|   stm32f427_437_429_439_wlcsp143 IBIS Model
[IBIS ver]   4.2
[File name]  stm32f427_437_429_439_wlcsp143.ibs
[File Rev]   1.3
[Date]   05-30-2014
[Source] Data Created at STMicroelectronics
[Notes]   File originated from ELDO simulations.
[Disclaimer]  This information is for modeling purpose only and is
   not guaranted. The information is subject to change without
   notice.
[Copyright] Copyright 2014 STMicroelectronics Inc.
[Component] stm32f427_437_429_439_wlcsp143
[Manufacturer] STMicroelectronics
[Package]
| variable   typ   min   max
R_pkg   0.0   NA   NA
L_pkg   0.0H   NA   NA
C_pkg   0.0F   NA   NA
[Pin]   signal_name   model_name  R_pin L_pin C_pin
A1   VDD  POWER
A10  PE1  io8p_arsudq_ft
A11  PDR_ON  io8p_arsudq_ft_v33
A2  PC10  io8p_arsudq_ft
A3  PD2  io8p_arsudq_ft
A4  PD5  io8p_arsudq_ft
A5  PD7  io8p_arsudq_ft
A6  PG12  io8p_arsudq_ft
A7  PG15  io8p_arsudq_ft
A8  PB6  io8p_arsudq_i2cin_ft
A9  PB8  io8p_arsudq_i2cin_ft
B1  PA14  io8p_arsudq_ft
B10  PE0  io8p_arsudq_ft
B11  PE4  io8p_arsudq_ft
B2  PC11  io8p_arsudq_ft
B3  PD0  io8p_arsudq_ft
B4  PD3  io8p_arsudq_ft
B5  PD4  io8p_arsudq_ft
B6  PG11  io8p_arsudq_ft
B7  PB3  io8p_arsudq_ft
B8  PB7  io8p_arsudq_i2cin_ft
B9  PB9  io8p_arsudq_i2cin_ft
C1  VDD  POWER
C10  PE3  io8p_arsudq_ft
C11  VBAT  POWER
C2  PA15  io8p_arsudq_ft
C3  PC12  io8p_arsudq_ft
C4  PD1  io8p_arsudq_ft
C5  VDD  POWER
C6  PG10  io8p_arsudq_ft
C7  PB4  io8p_arsudq_ft
C8  PB5  io8p_ar3wsudq_ft
C9  BOOT0  vpp_test_hv
D1   VCAP2  POWER
D10  PC13  io8p_arwsudq_ft_v33
D11  PC14  io8p_arwsudq_ft
D3  PA13  io8p_arsudq_ft
D4  PA11  io8usb_lsfs_otg_ft
D5  PA10  io8usb_id_otg_ft
D6  PG13  io8p_arsudq_ft
D7  VDD  POWER
D8  PE2  io8p_arsudq_ft
D9  PE5  io8p_arsudq_ft
E1  PA12  io8usb_lsfs_otg_ft
E10  VDD  POWER
E11  PC15  io8p_arsudq_ft
E2  PA9  io8usb_vbus_otg_ft
E3  PC9  io8p_arsudq_i2cin_ft
E4  PC8  io8p_arsudq_ft
E5  PG9  io8p_arsudq_ft
E6  VDD  POWER
E8  PE6  io8p_arsudq_ft
E9  PF1  io8p_arsudq_i2cin_ft
F1  PA8  io8p_arsudq_i2cin_ft
F10  PF2  io8p_arsudq_ft
F11  PF0  io8p_arsudq_i2cin_ft
F2  PC6  io8p_arsudq_ft
F3  PC7  io8p_arsudq_ft
F4  PD6  io8p_arsudq_ft
F6  PG14  io8p_arsudq_ft
F7  PF7  io8p_arwsudq_ft
F8  PF5  io8p_arwsudq_ft
F9  PF4  io8p_arwsudq_ft
G1  VDD  POWER
G10  PF6  io8p_arwsudq_ft
G11  PF3  io8p_arwsudq_ft
G2  PG8  io8p_arsudq_ft
G3  PG3  io8p_arsudq_ft
G4  PG6  io8p_arsudq_ft
G5  PG4  io8p_arsudq_ft
G6  PG5  io8p_arsudq_ft
G7  VDD  POWER
G8  PF9  io8p_arwsudq_ft
G9  PF10  io8p_arwsudq_ft
H1  PG7  io8p_arsudq_ft
H10  PH1  io8p_arsudq_ft
H11  PF8  io8p_arwsudq_ft
H4  PD10  io8p_arsudq_ft
H5  PD13  io8p_arsudq_ft
H6  PD12  io8p_arsudq_ft
H8  PC0  io8p_ar3wsudq_ft
H9  NRST  ioreset_ft_v33
J1  PG2  io8p_arsudq_ft
J10  PC2  io8p_ar3wsudq_ft
J11  PH0  io8p_arsudq_ft
J2  PD14  io8p_arsudq_ft
J3  PB15  io8usb_lsfs_otg_ft
J4  PE10  io8p_arsudq_ft
J5  VDD  POWER
J6  VDD  POWER
J7  VDD  POWER
J8  VDD  POWER
J9  PC3  io8p_ar3wsudq_ft_x2
K1   PD15  io8p_arsudq_ft
K10  VSSA  GND
| K11: io8p_combi = io8p_arsudq_ft_v33_c (PDR_ON) + io8p_ar3wsudq_ft_c (PC1)
K11  PC1   io8p_combi
K2  PD11  io8p_arsudq_ft
K3  PB14  io8usb_lsfs_otg_ft
K4  PE11  io8p_arsudq_ft
K5  PG1  io8p_arsudq_ft
K6  PF13  io8p_arsudq_ft
K7  PB1  io8p_ar3wsudq_ft
K8  PA1  io8p_ar3wsudq_ft
K9  PA0  io8p_ar3wsudq_ft_v33
L1   VDD  POWER
L10  VDDA  POWER
L11  VREF+  POWER
L2  PD8  io8p_arsudq_ft
L3  PE15  io8p_ar3wsudq_ft
L4  PE12  io8p_arsudq_ft
L5  PE7  io8p_arsudq_ft
L6  PF14  io8p_arsudq_ft
L7  PB2  io8p_ar3wsudq_ft
L8  PA7  io8p_ar3wsudq_ft
L9  PA2  io8p_ar3wsudq_ft
M1  PD9  io8p_arsudq_ft
M10  PA4  io8p_ar3wsudq_ft
M11  PA3  io8p_ar3wsudq_ft
M2  PB12  io8usb_id_otg_ft
M3  PB10  io8p_arsudq_i2cin_ft
M4  PE14  io8p_arsudq_ft
M5  PE8  io8p_arsudq_ft
M6  PF15  io8p_arsudq_ft
M7  PF11  io8p_arsudq_ft
M8  PC4  io8p_ar3wsudq_ft
M9  PA5  io8p_ar3wsudq_ft
N1  PB13  io8usb_vbus_otg_ft
N10  PA6  io8p_ar3wsudq_ft
N11  BYPASS_REG  io8p_arsudq_ft_v33
N2  VCAP1  POWER
N3  PB11  io8p_arsudq_i2cin_ft
N4  PE13  io8p_arsudq_ft
N5  PE9  io8p_arsudq_ft
N6  PG0  io8p_arsudq_ft
N7  PF12  io8p_arsudq_ft
N8  PB0  io8p_ar3wsudq_ft
N9  PC5  io8p_ar3wsudq_ft
[Diff Pin]   inv_pin   vdiff   tdelay_typ  tdelay_min  tdelay_max
D4   E1   200mV   NA   NA   NA
K1   J3   200mV   NA   NA   NA
[Model Selector] io8p_ar3wsudq_ft
io8p00_ar3wsudq_ft_pd_lv  "SPEED00 1P8V, PD=40kOhm"
io8p00_ar3wsudq_ft_pu_lv  "SPEED00 1P8V, PU=40kOhm"
io8p00_ar3wsudq_ft_lv  "SPEED00 1P8V"
io8p01_ar3wsudq_ft_pd_lv  "SPEED01 1P8V, PD=40kOhm"
io8p01_ar3wsudq_ft_pu_lv  "SPEED01 1P8V, PU=40kOhm"
io8p01_ar3wsudq_ft_lv  "SPEED01 1P8V"
io8p10_ar3wsudq_ft_pd_lv  "SPEED10 1P8V, PD=40kOhm"
io8p10_ar3wsudq_ft_pu_lv  "SPEED10 1P8V, PU=40kOhm"
io8p10_ar3wsudq_ft_lv  "SPEED10 1P8V"
io8p11_ar3wsudq_ft_pd_lv  "SPEED11 1P8V, PD=40kOhm"
io8p11_ar3wsudq_ft_pu_lv  "SPEED11 1P8V, PU=40kOhm"
io8p11_ar3wsudq_ft_lv  "SPEED11 1P8V"
io8p00_ar3wsudq_ft_pd  "SPEED00, PD=40kOhm"
io8p00_ar3wsudq_ft_pu  "SPEED00, PU=40kOhm"
io8p00_ar3wsudq_ft  "SPEED00"
io8p01_ar3wsudq_ft_pd  "SPEED01, PD=40kOhm"
io8p01_ar3wsudq_ft_pu  "SPEED01, PU=40kOhm"
io8p01_ar3wsudq_ft  "SPEED01"
io8p10_ar3wsudq_ft_pd  "SPEED10, PD=40kOhm"
io8p10_ar3wsudq_ft_pu  "SPEED10, PU=40kOhm"
io8p10_ar3wsudq_ft  "SPEED10"
io8p11_ar3wsudq_ft_pd  "SPEED11, PD=40kOhm"
io8p11_ar3wsudq_ft_pu  "SPEED11, PU=40kOhm"
io8p11_ar3wsudq_ft  "SPEED11"
[Model Selector] io8p_ar3wsudq_ft_v33
io8p00_ar3wsudq_ft_v33_pd_lv  "SPEED00 1P8V, PD=40kOhm"
io8p00_ar3wsudq_ft_v33_pu_lv  "SPEED00 1P8V, PU=40kOhm"
io8p00_ar3wsudq_ft_v33_lv  "SPEED00 1P8V"
io8p01_ar3wsudq_ft_v33_pd_lv  "SPEED01 1P8V, PD=40kOhm"
io8p01_ar3wsudq_ft_v33_pu_lv  "SPEED01 1P8V, PU=40kOhm"
io8p01_ar3wsudq_ft_v33_lv  "SPEED01 1P8V"
io8p10_ar3wsudq_ft_v33_pd_lv  "SPEED10 1P8V, PD=40kOhm"
io8p10_ar3wsudq_ft_v33_pu_lv  "SPEED10 1P8V, PU=40kOhm"
io8p10_ar3wsudq_ft_v33_lv  "SPEED10 1P8V"
io8p11_ar3wsudq_ft_v33_pd_lv  "SPEED11 1P8V, PD=40kOhm"
io8p11_ar3wsudq_ft_v33_pu_lv  "SPEED11 1P8V, PU=40kOhm"
io8p11_ar3wsudq_ft_v33_lv  "SPEED11 1P8V"
io8p00_ar3wsudq_ft_v33_pd  "SPEED00, PD=40kOhm"
io8p00_ar3wsudq_ft_v33_pu  "SPEED00, PU=40kOhm"
io8p00_ar3wsudq_ft_v33  "SPEED00"
io8p01_ar3wsudq_ft_v33_pd  "SPEED01, PD=40kOhm"
io8p01_ar3wsudq_ft_v33_pu  "SPEED01, PU=40kOhm"
io8p01_ar3wsudq_ft_v33  "SPEED01"
io8p10_ar3wsudq_ft_v33_pd  "SPEED10, PD=40kOhm"
io8p10_ar3wsudq_ft_v33_pu  "SPEED10, PU=40kOhm"
io8p10_ar3wsudq_ft_v33  "SPEED10"
io8p11_ar3wsudq_ft_v33_pd  "SPEED11, PD=40kOhm"
io8p11_ar3wsudq_ft_v33_pu  "SPEED11, PU=40kOhm"
io8p11_ar3wsudq_ft_v33  "SPEED11"
[Model Selector] io8p_arsudq_ft
io8p00_arsudq_ft_pd_lv  "SPEED00 1P8V, PD=40kOhm"
io8p00_arsudq_ft_pu_lv  "SPEED00 1P8V, PU=40kOhm"
io8p00_arsudq_ft_lv  "SPEED00 1P8V"
io8p01_arsudq_ft_pd_lv  "SPEED01 1P8V, PD=40kOhm"
io8p01_arsudq_ft_pu_lv  "SPEED01 1P8V, PU=40kOhm"
io8p01_arsudq_ft_lv  "SPEED01 1P8V"
io8p10_arsudq_ft_pd_lv  "SPEED10 1P8V, PD=40kOhm"
io8p10_arsudq_ft_pu_lv  "SPEED10 1P8V, PU=40kOhm"
io8p10_arsudq_ft_lv  "SPEED10 1P8V"
io8p11_arsudq_ft_pd_lv  "SPEED11 1P8V, PD=40kOhm"
io8p11_arsudq_ft_pu_lv  "SPEED11 1P8V, PU=40kOhm"
io8p11_arsudq_ft_lv  "SPEED11 1P8V"
io8p00_arsudq_ft_pd  "SPEED00, PD=40kOhm"
io8p00_arsudq_ft_pu  "SPEED00, PU=40kOhm"
io8p00_arsudq_ft  "SPEED00"
io8p01_arsudq_ft_pd  "SPEED01, PD=40kOhm"
io8p01_arsudq_ft_pu  "SPEED01, PU=40kOhm"
io8p01_arsudq_ft  "SPEED01"
io8p10_arsudq_ft_pd  "SPEED10, PD=40kOhm"
io8p10_arsudq_ft_pu  "SPEED10, PU=40kOhm"
io8p10_arsudq_ft  "SPEED10"
io8p11_arsudq_ft_pd  "SPEED11, PD=40kOhm"
io8p11_arsudq_ft_pu  "SPEED11, PU=40kOhm"
io8p11_arsudq_ft  "SPEED11"
[Model Selector] io8p_arsudq_ft_v33
io8p00_arsudq_ft_v33_pd_lv  "SPEED00 1P8V, PD=40kOhm"
io8p00_arsudq_ft_v33_pu_lv  "SPEED00 1P8V, PU=40kOhm"
io8p00_arsudq_ft_v33_lv  "SPEED00 1P8V"
io8p01_arsudq_ft_v33_pd_lv  "SPEED01 1P8V, PD=40kOhm"
io8p01_arsudq_ft_v33_pu_lv  "SPEED01 1P8V, PU=40kOhm"
io8p01_arsudq_ft_v33_lv  "SPEED01 1P8V"
io8p10_arsudq_ft_v33_pd_lv  "SPEED10 1P8V, PD=40kOhm"
io8p10_arsudq_ft_v33_pu_lv  "SPEED10 1P8V, PU=40kOhm"
io8p10_arsudq_ft_v33_lv  "SPEED10 1P8V"
io8p11_arsudq_ft_v33_pd_lv  "SPEED11 1P8V, PD=40kOhm"
io8p11_arsudq_ft_v33_pu_lv  "SPEED11 1P8V, PU=40kOhm"
io8p11_arsudq_ft_v33_lv  "SPEED11 1P8V"
io8p00_arsudq_ft_v33_pd  "SPEED00, PD=40kOhm"
io8p00_arsudq_ft_v33_pu  "SPEED00, PU=40kOhm"
io8p00_arsudq_ft_v33  "SPEED00"
io8p01_arsudq_ft_v33_pd  "SPEED01, PD=40kOhm"
io8p01_arsudq_ft_v33_pu  "SPEED01, PU=40kOhm"
io8p01_arsudq_ft_v33  "SPEED01"
io8p10_arsudq_ft_v33_pd  "SPEED10, PD=40kOhm"
io8p10_arsudq_ft_v33_pu  "SPEED10, PU=40kOhm"
io8p10_arsudq_ft_v33  "SPEED10"
io8p11_arsudq_ft_v33_pd  "SPEED11, PD=40kOhm"
io8p11_arsudq_ft_v33_pu  "SPEED11, PU=40kOhm"
io8p11_arsudq_ft_v33  "SPEED11"
[Model Selector] io8p_arsudq_i2cin_ft
io8p00_arsudq_i2cin_ft_pd_lv  "SPEED00 1P8V, PD=40kOhm"
io8p00_arsudq_i2cin_ft_pu_lv  "SPEED00 1P8V, PU=40kOhm"
io8p00_arsudq_i2cin_ft_lv  "SPEED00 1P8V"
io8p01_arsudq_i2cin_ft_pd_lv  "SPEED01 1P8V, PD=40kOhm"
io8p01_arsudq_i2cin_ft_pu_lv  "SPEED01 1P8V, PU=40kOhm"
io8p01_arsudq_i2cin_ft_lv  "SPEED01 1P8V"
io8p10_arsudq_i2cin_ft_pd_lv  "SPEED10 1P8V, PD=40kOhm"
io8p10_arsudq_i2cin_ft_pu_lv  "SPEED10 1P8V, PU=40kOhm"
io8p10_arsudq_i2cin_ft_lv  "SPEED10 1P8V"
io8p11_arsudq_i2cin_ft_pd_lv  "SPEED11 1P8V, PD=40kOhm"
io8p11_arsudq_i2cin_ft_pu_lv  "SPEED11 1P8V, PU=40kOhm"
io8p11_arsudq_i2cin_ft_lv  "SPEED11 1P8V"
io8p00_arsudq_i2cin_ft_pd  "SPEED00, PD=40kOhm"
io8p00_arsudq_i2cin_ft_pu  "SPEED00, PU=40kOhm"
io8p00_arsudq_i2cin_ft  "SPEED00"
io8p01_arsudq_i2cin_ft_pd  "SPEED01, PD=40kOhm"
io8p01_arsudq_i2cin_ft_pu  "SPEED01, PU=40kOhm"
io8p01_arsudq_i2cin_ft  "SPEED01"
io8p10_arsudq_i2cin_ft_pd  "SPEED10, PD=40kOhm"
io8p10_arsudq_i2cin_ft_pu  "SPEED10, PU=40kOhm"
io8p10_arsudq_i2cin_ft  "SPEED10"
io8p11_arsudq_i2cin_ft_pd  "SPEED11, PD=40kOhm"
io8p11_arsudq_i2cin_ft_pu  "SPEED11, PU=40kOhm"
io8p11_arsudq_i2cin_ft  "SPEED11"
[Model Selector] io8p_arwsudq_ft
io8p00_arwsudq_ft_pd_lv  "SPEED00 1P8V, PD=40kOhm"
io8p00_arwsudq_ft_pu_lv  "SPEED00 1P8V, PU=40kOhm"
io8p00_arwsudq_ft_lv  "SPEED00 1P8V"
io8p01_arwsudq_ft_pd_lv  "SPEED01 1P8V, PD=40kOhm"
io8p01_arwsudq_ft_pu_lv  "SPEED01 1P8V, PU=40kOhm"
io8p01_arwsudq_ft_lv  "SPEED01 1P8V"
io8p10_arwsudq_ft_pd_lv  "SPEED10 1P8V, PD=40kOhm"
io8p10_arwsudq_ft_pu_lv  "SPEED10 1P8V, PU=40kOhm"
io8p10_arwsudq_ft_lv  "SPEED10 1P8V"
io8p11_arwsudq_ft_pd_lv  "SPEED11 1P8V, PD=40kOhm"
io8p11_arwsudq_ft_pu_lv  "SPEED11 1P8V, PU=40kOhm"
io8p11_arwsudq_ft_lv  "SPEED11 1P8V"
io8p00_arwsudq_ft_pd  "SPEED00, PD=40kOhm"
io8p00_arwsudq_ft_pu  "SPEED00, PU=40kOhm"
io8p00_arwsudq_ft  "SPEED00"
io8p01_arwsudq_ft_pd  "SPEED01, PD=40kOhm"
io8p01_arwsudq_ft_pu  "SPEED01, PU=40kOhm"
io8p01_arwsudq_ft  "SPEED01"
io8p10_arwsudq_ft_pd  "SPEED10, PD=40kOhm"
io8p10_arwsudq_ft_pu  "SPEED10, PU=40kOhm"
io8p10_arwsudq_ft  "SPEED10"
io8p11_arwsudq_ft_pd  "SPEED11, PD=40kOhm"
io8p11_arwsudq_ft_pu  "SPEED11, PU=40kOhm"
io8p11_arwsudq_ft  "SPEED11"
[Model Selector] io8p_arwsudq_ft_v33
io8p00_arwsudq_ft_v33_pd_lv  "SPEED00 1P8V, PD=40kOhm"
io8p00_arwsudq_ft_v33_pu_lv  "SPEED00 1P8V, PU=40kOhm"
io8p00_arwsudq_ft_v33_lv  "SPEED00 1P8V"
io8p01_arwsudq_ft_v33_pd_lv  "SPEED01 1P8V, PD=40kOhm"
io8p01_arwsudq_ft_v33_pu_lv  "SPEED01 1P8V, PU=40kOhm"
io8p01_arwsudq_ft_v33_lv  "SPEED01 1P8V"
io8p10_arwsudq_ft_v33_pd_lv  "SPEED10 1P8V, PD=40kOhm"
io8p10_arwsudq_ft_v33_pu_lv  "SPEED10 1P8V, PU=40kOhm"
io8p10_arwsudq_ft_v33_lv  "SPEED10 1P8V"
io8p11_arwsudq_ft_v33_pd_lv  "SPEED11 1P8V, PD=40kOhm"
io8p11_arwsudq_ft_v33_pu_lv  "SPEED11 1P8V, PU=40kOhm"
io8p11_arwsudq_ft_v33_lv  "SPEED11 1P8V"
io8p00_arwsudq_ft_v33_pd  "SPEED00, PD=40kOhm"
io8p00_arwsudq_ft_v33_pu  "SPEED00, PU=40kOhm"
io8p00_arwsudq_ft_v33  "SPEED00"
io8p01_arwsudq_ft_v33_pd  "SPEED01, PD=40kOhm"
io8p01_arwsudq_ft_v33_pu  "SPEED01, PU=40kOhm"
io8p01_arwsudq_ft_v33  "SPEED01"
io8p10_arwsudq_ft_v33_pd  "SPEED10, PD=40kOhm"
io8p10_arwsudq_ft_v33_pu  "SPEED10, PU=40kOhm"
io8p10_arwsudq_ft_v33  "SPEED10"
io8p11_arwsudq_ft_v33_pd  "SPEED11, PD=40kOhm"
io8p11_arwsudq_ft_v33_pu  "SPEED11, PU=40kOhm"
io8p11_arwsudq_ft_v33  "SPEED11"
[Model Selector] io8usb_id_otg_ft
io8p00_id_otg_ft_pd_lv  "SPEED00 1P8V, PD=14kOhm"
io8p00_id_otg_ft_pu_lv  "SPEED00 1P8V, PU=14kOhm"
io8p00_id_otg_ft_lv  "SPEED00 1P8V"
io8p01_id_otg_ft_pd_lv  "SPEED01 1P8V, PD=14kOhm"
io8p01_id_otg_ft_pu_lv  "SPEED01 1P8V, PU=14kOhm"
io8p01_id_otg_ft_lv  "SPEED01 1P8V"
io8p10_id_otg_ft_pd_lv  "SPEED10 1P8V, PD=14kOhm"
io8p10_id_otg_ft_pu_lv  "SPEED10 1P8V, PU=14kOhm"
io8p10_id_otg_ft_lv  "SPEED10 1P8V"
io8p11_id_otg_ft_pd_lv  "SPEED11 1P8V, PD=14kOhm"
io8p11_id_otg_ft_pu_lv  "SPEED11 1P8V, PU=14kOhm"
io8p11_id_otg_ft_lv  "SPEED11 1P8V"
io8p00_id_otg_ft_pd  "SPEED00, PD=14kOhm"
io8p00_id_otg_ft_pu  "SPEED00, PU=14kOhm"
io8p00_id_otg_ft  "SPEED00"
io8p01_id_otg_ft_pd  "SPEED01, PD=14kOhm"
io8p01_id_otg_ft_pu  "SPEED01, PU=14kOhm"
io8p01_id_otg_ft  "SPEED01"
io8p10_id_otg_ft_pd  "SPEED10, PD=14kOhm"
io8p10_id_otg_ft_pu  "SPEED10, PU=14kOhm"
io8p10_id_otg_ft  "SPEED10"
io8p11_id_otg_ft_pd  "SPEED11, PD=14kOhm"
io8p11_id_otg_ft_pu  "SPEED11, PU=14kOhm"
io8p11_id_otg_ft  "SPEED11"
[Model Selector] io8usb_lsfs_otg_ft
io8usb_ls_otg_ft_dpdn_pd  "LS USB DP/DN IO + PD=20kOhm"
io8usb_ls_otg_ft_dpdn_pupu2  "LS USB DP/DN IO + PU/PU2=2.2kOhm"
io8usb_ls_otg_ft_dpdn_pu2  "LS USB DP/DN IO + PU2=1.2kOhm"
io8usb_ls_otg_ft_dpdn_pu  "LS USB DP/DN IO + PU=1.2kOhm"
io8usb_ls_otg_ft_dpdn  "LS USB DP/DN IO"
io8usb_fs_otg_ft_dpdn_pd  "HS USB DP/DN IO + PD=20kOhm"
io8usb_fs_otg_ft_dpdn_pupu2  "HS USB DP/DN IO + PU/PU2=2.2kOhm"
io8usb_fs_otg_ft_dpdn_pu2  "HS USB DP/DN IO + PU2=1.2kOhm"
io8usb_fs_otg_ft_dpdn_pu  "HS USB DP/DN IO + PU=1.2kOhm"
io8usb_fs_otg_ft_dpdn  "HS USB DP/DN IO"
io8p00_lsfs_otg_ft_pd_lv  "SPEED00 1P8V, PD=40kOhm"
io8p00_lsfs_otg_ft_pu_lv  "SPEED00 1P8V, PU=40kOhm"
io8p00_lsfs_otg_ft_lv  "SPEED00 1P8V"
io8p01_lsfs_otg_ft_pd_lv  "SPEED01 1P8V, PD=40kOhm"
io8p01_lsfs_otg_ft_pu_lv  "SPEED01 1P8V, PU=40kOhm"
io8p01_lsfs_otg_ft_lv  "SPEED01 1P8V"
io8p10_lsfs_otg_ft_pd_lv  "SPEED10 1P8V, PD=40kOhm"
io8p10_lsfs_otg_ft_pu_lv  "SPEED10 1P8V, PU=40kOhm"
io8p10_lsfs_otg_ft_lv  "SPEED10 1P8V"
io8p11_lsfs_otg_ft_pd_lv  "SPEED11 1P8V, PD=40kOhm"
io8p11_lsfs_otg_ft_pu_lv  "SPEED11 1P8V, PU=40kOhm"
io8p11_lsfs_otg_ft_lv  "SPEED11 1P8V"
io8p00_lsfs_otg_ft_pd  "SPEED00, PD=40kOhm"
io8p00_lsfs_otg_ft_pu  "SPEED00, PU=40kOhm"
io8p00_lsfs_otg_ft  "SPEED00"
io8p01_lsfs_otg_ft_pd  "SPEED01, PD=40kOhm"
io8p01_lsfs_otg_ft_pu  "SPEED01, PU=40kOhm"
io8p01_lsfs_otg_ft  "SPEED01"
io8p10_lsfs_otg_ft_pd  "SPEED10, PD=40kOhm"
io8p10_lsfs_otg_ft_pu  "SPEED10, PU=40kOhm"
io8p10_lsfs_otg_ft  "SPEED10"
io8p11_lsfs_otg_ft_pd  "SPEED11, PD=40kOhm"
io8p11_lsfs_otg_ft_pu  "SPEED11, PU=40kOhm"
io8p11_lsfs_otg_ft  "SPEED11"
[Model Selector] io8usb_vbus_otg_ft
io8psenb_vbus_otg_ft  "VBUS PULSE, SENSE VB"
io8psenab_vbus_otg_ft  "VBUS PULSE, SENSE VA and VB"
io8psena_vbus_otg_ft  "VBUS PULSE, SENSE VA"
io8psen_vbus_otg_ft  "VBUS PULSE"
io8p00_vbus_otg_ft_pd_lv  "SPEED00 1P8V, PD=40kOhm"
io8p00_vbus_otg_ft_pu_lv  "SPEED00 1P8V, PU=40kOhm"
io8p00_vbus_otg_ft_lv  "SPEED00 1P8V"
io8p01_vbus_otg_ft_pd_lv  "SPEED01 1P8V, PD=40kOhm"
io8p01_vbus_otg_ft_pu_lv  "SPEED01 1P8V, PU=40kOhm"
io8p01_vbus_otg_ft_lv  "SPEED01 1P8V"
io8p10_vbus_otg_ft_pd_lv  "SPEED10 1P8V, PD=40kOhm"
io8p10_vbus_otg_ft_pu_lv  "SPEED10 1P8V, PU=40kOhm"
io8p10_vbus_otg_ft_lv  "SPEED10 1P8V"
io8p11_vbus_otg_ft_pd_lv  "SPEED11 1P8V, PD=40kOhm"
io8p11_vbus_otg_ft_pu_lv  "SPEED11 1P8V, PU=40kOhm"
io8p11_vbus_otg_ft_lv  "SPEED11 1P8V"
io8p00_vbus_otg_ft_pd  "SPEED00, PD=40kOhm"
io8p00_vbus_otg_ft_pu  "SPEED00, PU=40kOhm"
io8p00_vbus_otg_ft  "SPEED00"
io8p01_vbus_otg_ft_pd  "SPEED01, PD=40kOhm"
io8p01_vbus_otg_ft_pu  "SPEED01, PU=40kOhm"
io8p01_vbus_otg_ft  "SPEED01"
io8p10_vbus_otg_ft_pd  "SPEED10, PD=40kOhm"
io8p10_vbus_otg_ft_pu  "SPEED10, PU=40kOhm"
io8p10_vbus_otg_ft  "SPEED10"
io8p11_vbus_otg_ft_pd  "SPEED11, PD=40kOhm"
io8p11_vbus_otg_ft_pu  "SPEED11, PU=40kOhm"
io8p11_vbus_otg_ft  "SPEED11"
[Model Selector] ioreset_ft_v33
ioreset_ft_v33_pu_lv  "IORESET 1P8V + PU=40kOhm"
ioreset_ft_v33_nopu_lv  "IORESET 1P8V"
ioreset_ft_v33_pu  "IORESET + PU=40kOhm"
ioreset_ft_v33_nopu  "IORESET"
[Model Selector] io8p_ar3wsudq_ft_x2
io8p00_ar3wsudq_ft_x2_pd_lv  "SPEED00 1P8V, PD=40kOhm"
io8p00_ar3wsudq_ft_x2_pu_lv  "SPEED00 1P8V, PU=40kOhm"
io8p00_ar3wsudq_ft_x2_lv  "SPEED00 1P8V"
io8p01_ar3wsudq_ft_x2_pd_lv  "SPEED01 1P8V, PD=40kOhm"
io8p01_ar3wsudq_ft_x2_pu_lv  "SPEED01 1P8V, PU=40kOhm"
io8p01_ar3wsudq_ft_x2_lv  "SPEED01 1P8V"
io8p10_ar3wsudq_ft_x2_pd_lv  "SPEED10 1P8V, PD=40kOhm"
io8p10_ar3wsudq_ft_x2_pu_lv  "SPEED10 1P8V, PU=40kOhm"
io8p10_ar3wsudq_ft_x2_lv  "SPEED10 1P8V"
io8p11_ar3wsudq_ft_x2_pd_lv  "SPEED11 1P8V, PD=40kOhm"
io8p11_ar3wsudq_ft_x2_pu_lv  "SPEED11 1P8V, PU=40kOhm"
io8p11_ar3wsudq_ft_x2_lv  "SPEED11 1P8V"
io8p00_ar3wsudq_ft_x2_pd  "SPEED00, PD=40kOhm"
io8p00_ar3wsudq_ft_x2_pu  "SPEED00, PU=40kOhm"
io8p00_ar3wsudq_ft_x2  "SPEED00"
io8p01_ar3wsudq_ft_x2_pd  "SPEED01, PD=40kOhm"
io8p01_ar3wsudq_ft_x2_pu  "SPEED01, PU=40kOhm"
io8p01_ar3wsudq_ft_x2  "SPEED01"
io8p10_ar3wsudq_ft_x2_pd  "SPEED10, PD=40kOhm"
io8p10_ar3wsudq_ft_x2_pu  "SPEED10, PU=40kOhm"
io8p10_ar3wsudq_ft_x2  "SPEED10"
io8p11_ar3wsudq_ft_x2_pd  "SPEED11, PD=40kOhm"
io8p11_ar3wsudq_ft_x2_pu  "SPEED11, PU=40kOhm"
io8p11_ar3wsudq_ft_x2  "SPEED11"
[Model Selector] io8p_combi
| Sub model: [Model Selector] io8p_arsudq_ft_v33_c
io8p00_arsudq_ft_v33_c_pd_lv  "signal PDR_ON, SPEED00 1P8V, PD=40kOhm"
io8p00_arsudq_ft_v33_c_pu_lv  "signal PDR_ON, SPEED00 1P8V, PU=40kOhm"
io8p00_arsudq_ft_v33_c_lv  "signal PDR_ON, SPEED00 1P8V"
io8p01_arsudq_ft_v33_c_pd_lv  "signal PDR_ON, SPEED01 1P8V, PD=40kOhm"
io8p01_arsudq_ft_v33_c_pu_lv  "signal PDR_ON, SPEED01 1P8V, PU=40kOhm"
io8p01_arsudq_ft_v33_c_lv  "signal PDR_ON, SPEED01 1P8V"
io8p10_arsudq_ft_v33_c_pd_lv  "signal PDR_ON, SPEED10 1P8V, PD=40kOhm"
io8p10_arsudq_ft_v33_c_pu_lv  "signal PDR_ON, SPEED10 1P8V, PU=40kOhm"
io8p10_arsudq_ft_v33_c_lv  "signal PDR_ON, SPEED10 1P8V"
io8p11_arsudq_ft_v33_c_pd_lv  "signal PDR_ON, SPEED11 1P8V, PD=40kOhm"
io8p11_arsudq_ft_v33_c_pu_lv  "signal PDR_ON, SPEED11 1P8V, PU=40kOhm"
io8p11_arsudq_ft_v33_c_lv  "signal PDR_ON, SPEED11 1P8V"
io8p00_arsudq_ft_v33_c_pd  "signal PDR_ON, SPEED00, PD=40kOhm"
io8p00_arsudq_ft_v33_c_pu  "signal PDR_ON, SPEED00, PU=40kOhm"
io8p00_arsudq_ft_v33_c  "signal PDR_ON, SPEED00"
io8p01_arsudq_ft_v33_c_pd  "signal PDR_ON, SPEED01, PD=40kOhm"
io8p01_arsudq_ft_v33_c_pu  "signal PDR_ON, SPEED01, PU=40kOhm"
io8p01_arsudq_ft_v33_c  "signal PDR_ON, SPEED01"
io8p10_arsudq_ft_v33_c_pd  "signal PDR_ON, SPEED10, PD=40kOhm"
io8p10_arsudq_ft_v33_c_pu  "signal PDR_ON, SPEED10, PU=40kOhm"
io8p10_arsudq_ft_v33_c  "signal PDR_ON, SPEED10"
io8p11_arsudq_ft_v33_c_pd  "signal PDR_ON, SPEED11, PD=40kOhm"
io8p11_arsudq_ft_v33_c_pu  "signal PDR_ON, SPEED11, PU=40kOhm"
io8p11_arsudq_ft_v33_c  "signal PDR_ON, SPEED11"
| Sub model: [Model Selector] io8p_ar3wsudq_ft_c
io8p00_ar3wsudq_ft_c_pd_lv  "signal PC1, SPEED00 1P8V, PD=40kOhm"
io8p00_ar3wsudq_ft_c_pu_lv  "signal PC1, SPEED00 1P8V, PU=40kOhm"
io8p00_ar3wsudq_ft_c_lv  "signal PC1, SPEED00 1P8V"
io8p01_ar3wsudq_ft_c_pd_lv  "signal PC1, SPEED01 1P8V, PD=40kOhm"
io8p01_ar3wsudq_ft_c_pu_lv  "signal PC1, SPEED01 1P8V, PU=40kOhm"
io8p01_ar3wsudq_ft_c_lv  "signal PC1, SPEED01 1P8V"
io8p10_ar3wsudq_ft_c_pd_lv  "signal PC1, SPEED10 1P8V, PD=40kOhm"
io8p10_ar3wsudq_ft_c_pu_lv  "signal PC1, SPEED10 1P8V, PU=40kOhm"
io8p10_ar3wsudq_ft_c_lv  "signal PC1, SPEED10 1P8V"
io8p11_ar3wsudq_ft_c_pd_lv  "signal PC1, SPEED11 1P8V, PD=40kOhm"
io8p11_ar3wsudq_ft_c_pu_lv  "signal PC1, SPEED11 1P8V, PU=40kOhm"
io8p11_ar3wsudq_ft_c_lv  "signal PC1, SPEED11 1P8V"
io8p00_ar3wsudq_ft_c_pd  "signal PC1, SPEED00, PD=40kOhm"
io8p00_ar3wsudq_ft_c_pu  "signal PC1, SPEED00, PU=40kOhm"
io8p00_ar3wsudq_ft_c  "signal PC1, SPEED00"
io8p01_ar3wsudq_ft_c_pd  "signal PC1, SPEED01, PD=40kOhm"
io8p01_ar3wsudq_ft_c_pu  "signal PC1, SPEED01, PU=40kOhm"
io8p01_ar3wsudq_ft_c  "signal PC1, SPEED01"
io8p10_ar3wsudq_ft_c_pd  "signal PC1, SPEED10, PD=40kOhm"
io8p10_ar3wsudq_ft_c_pu  "signal PC1, SPEED10, PU=40kOhm"
io8p10_ar3wsudq_ft_c  "signal PC1, SPEED10"
io8p11_ar3wsudq_ft_c_pd  "signal PC1, SPEED11, PD=40kOhm"
io8p11_ar3wsudq_ft_c_pu  "signal PC1, SPEED11, PU=40kOhm"
io8p11_ar3wsudq_ft_c  "signal PC1, SPEED11"
[Model Selector] vpp_test_hv
vpp_test_hv_2p4  "Input Buffer 1P8V"
vpp_test_hv_3p3  "Input Buffer"
| Models and submodels in the file (332): io8p00_ar3wsudq_ft_pd_lv (I/O), io8p00_ar3wsudq_ft_pu_lv (I/O), io8p00_ar3wsudq_ft_lv (I/O), io8p01_ar3wsudq_ft_pd_lv (I/O), io8p01_ar3wsudq_ft_pu_lv (I/O), io8p01_ar3wsudq_ft_lv (I/O), io8p10_ar3wsudq_ft_pd_lv (I/O), io8p10_ar3wsudq_ft_pu_lv (I/O), io8p10_ar3wsudq_ft_lv (I/O), io8p11_ar3wsudq_ft_pd_lv (I/O), io8p11_ar3wsudq_ft_pu_lv (I/O), io8p11_ar3wsudq_ft_lv (I/O), io8p00_ar3wsudq_ft_pd (I/O), io8p00_ar3wsudq_ft_pu (I/O), io8p00_ar3wsudq_ft (I/O), io8p01_ar3wsudq_ft_pd (I/O), io8p01_ar3wsudq_ft_pu (I/O), io8p01_ar3wsudq_ft (I/O), io8p10_ar3wsudq_ft_pd (I/O), io8p10_ar3wsudq_ft_pu (I/O), io8p10_ar3wsudq_ft (I/O), io8p11_ar3wsudq_ft_pd (I/O), io8p11_ar3wsudq_ft_pu (I/O), io8p11_ar3wsudq_ft (I/O), io8p00_ar3wsudq_ft_v33_pd_lv (I/O), io8p00_ar3wsudq_ft_v33_pu_lv (I/O), io8p00_ar3wsudq_ft_v33_lv (I/O), io8p01_ar3wsudq_ft_v33_pd_lv (I/O), io8p01_ar3wsudq_ft_v33_pu_lv (I/O), io8p01_ar3wsudq_ft_v33_lv (I/O), io8p10_ar3wsudq_ft_v33_pd_lv (I/O), io8p10_ar3wsudq_ft_v33_pu_lv (I/O), io8p10_ar3wsudq_ft_v33_lv (I/O), io8p11_ar3wsudq_ft_v33_pd_lv (I/O), io8p11_ar3wsudq_ft_v33_pu_lv (I/O), io8p11_ar3wsudq_ft_v33_lv (I/O), io8p00_ar3wsudq_ft_v33_pd (I/O), io8p00_ar3wsudq_ft_v33_pu (I/O), io8p00_ar3wsudq_ft_v33 (I/O), io8p01_ar3wsudq_ft_v33_pd (I/O), io8p01_ar3wsudq_ft_v33_pu (I/O), io8p01_ar3wsudq_ft_v33 (I/O), io8p10_ar3wsudq_ft_v33_pd (I/O), io8p10_ar3wsudq_ft_v33_pu (I/O), io8p10_ar3wsudq_ft_v33 (I/O), io8p11_ar3wsudq_ft_v33_pd (I/O), io8p11_ar3wsudq_ft_v33_pu (I/O), io8p11_ar3wsudq_ft_v33 (I/O), io8p00_arsudq_ft_pd_lv (I/O), io8p00_arsudq_ft_pu_lv (I/O), io8p00_arsudq_ft_lv (I/O), io8p01_arsudq_ft_pd_lv (I/O), io8p01_arsudq_ft_pu_lv (I/O), io8p01_arsudq_ft_lv (I/O), io8p10_arsudq_ft_pd_lv (I/O), io8p10_arsudq_ft_pu_lv (I/O), io8p10_arsudq_ft_lv (I/O), io8p11_arsudq_ft_pd_lv (I/O), io8p11_arsudq_ft_pu_lv (I/O), io8p11_arsudq_ft_lv (I/O), io8p00_arsudq_ft_pd (I/O), io8p00_arsudq_ft_pu (I/O), io8p00_arsudq_ft (I/O), io8p01_arsudq_ft_pd (I/O), io8p01_arsudq_ft_pu (I/O), io8p01_arsudq_ft (I/O), io8p10_arsudq_ft_pd (I/O), io8p10_arsudq_ft_pu (I/O), io8p10_arsudq_ft (I/O), io8p11_arsudq_ft_pd (I/O), io8p11_arsudq_ft_pu (I/O), io8p11_arsudq_ft (I/O), io8p00_arsudq_ft_v33_pd_lv (I/O), io8p00_arsudq_ft_v33_pu_lv (I/O), io8p00_arsudq_ft_v33_lv (I/O), io8p01_arsudq_ft_v33_pd_lv (I/O), io8p01_arsudq_ft_v33_pu_lv (I/O), io8p01_arsudq_ft_v33_lv (I/O), io8p10_arsudq_ft_v33_pd_lv (I/O), io8p10_arsudq_ft_v33_pu_lv (I/O)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
